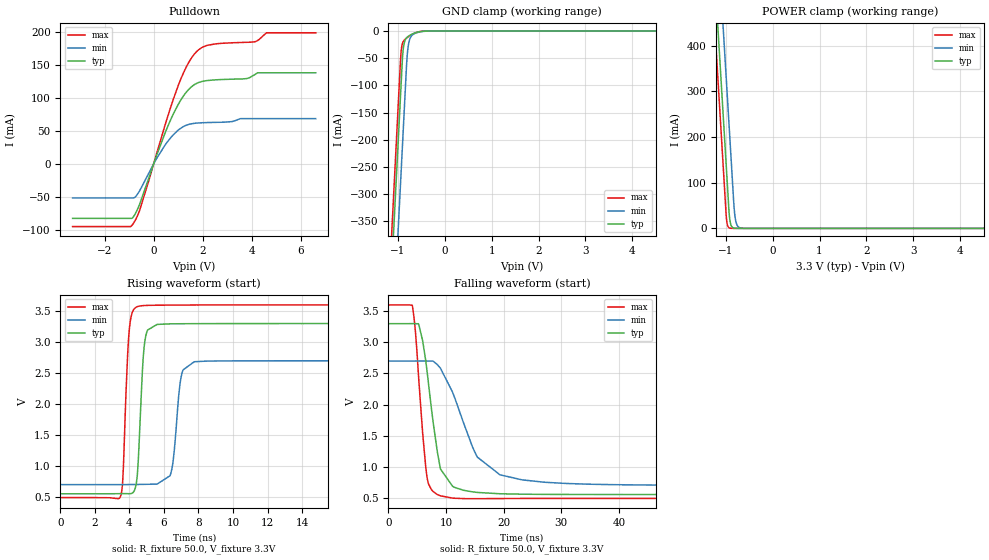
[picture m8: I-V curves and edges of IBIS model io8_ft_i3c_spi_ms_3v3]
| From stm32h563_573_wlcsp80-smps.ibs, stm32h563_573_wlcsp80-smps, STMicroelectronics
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[Model]   io8_ft_i3c_spi_ms_3v3
Model_type I/O_open_drain
Polarity   Non-Inverting
Enable   Active-Low
| CAP_THRESHOLD on pad IOFT is "UDTCAPC" :
| Rising=20.0% of vddiom   Falling=80.0% of vddiom
| C_comp min and max val. don't necessarily correlate with the min and max pvt
| but are the smallest and greatest pad capacitance found.
| var   typ   min   max
C_comp   3.95818pF  3.95032pF  4.00761pF
|C_comp_pulldown   3.95818pF  3.95032pF  4.00761pF
Vinl = 1.35V
Vinh = 1.8V
Vmeas = 1.65V   | Reference voltage for timing measurements
Cref  = 50.0pF   | Timing specification test load capacitance value
Rref  = 1.0MOhm   | Timing specification test load resistance value
Vref  = 1.815V   | Timing specification test load voltage
[Model Spec]
| TIME_THRESHOLD on pin ZII2CV11 is "CMOS" :
| Rising=40.0% of vdd   Falling=60.0% of vdd
Vinl 1.29880V 1.07480V 1.40680V
Vinh 1.77520V 1.49320V 1.89720V
| variable   typ   min   max
[Temperature Range] 25.0 125.0 -40.0
| variable   typ   min   max
[Voltage Range] 3.3V 2.7V 3.6V
| variable   typ   min   max
[POWER Clamp Reference] 3.3V 2.7V 3.6V
| variable   typ   min   max
[GND Clamp Reference] 0V 0V 0V
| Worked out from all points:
|   slope of the pulldown table from 0 to 0.495 V, typ, clamps not added: 10 ohm
|   GND clamp passes 1 mA (typ) near -0.52 V on its own axis
|   POWER clamp passes 1 mA (typ) near -0.84 V on its own axis
|   rising waveform, R_fixture 50.0, V_fixture 3.3V: 20-80 % time 285ps typ, 381ps min, 266ps max; typ from 0.556 V to 3.3 V
|   falling waveform, R_fixture 50.0, V_fixture 3.3V: 20-80 % time 2.35ns typ, 5.6ns min, 1.51ns max; typ from 3.3 V to 0.556 V
[POWER Clamp]
-3.3V     4.068A     4.259A     3.957A
-1.25V    582.8mA    774.2mA    471.5mA
-1.21V    514.8mA    706.2mA    403.5mA
-1.13V    378.8mA    570.2mA    267.5mA
-1.04V    225.8mA    417.2mA    114.5mA
-980mV    123.8mA    315.2mA    17.95mA
-920mV    26.3mA     213.2mA    906uA
-880mV    5.543mA    145.2mA    123.7uA
-810mV    363.5uA    33.6mA     3.798uA
-770mV    76.62uA    10.47mA    519.4nA
-690mV    3.409uA    1.017mA    10.46nA
6.6V      0A         0A         0A
[GND Clamp]
-3.3V     -4.13A     -4.291A    -4.063A
-1.25V    -644.7mA   -806.4mA   -578.1mA
-940mV    -117.7mA   -279.4mA   -51.06mA
-920mV    -83.75mA   -245.4mA   -31.43mA
-900mV    -50.5mA    -211.4mA   -23.14mA
-880mV    -31.27mA   -177.4mA   -19.1mA
-850mV    -18.68mA   -126.4mA   -15.73mA
-800mV    -11.46mA   -46.4mA    -12.03mA
-760mV    -8.752mA   -20.02mA   -9.606mA
-680mV    -5.122mA   -6.673mA   -5.579mA
-300mV    -5.379uA   -47.63uA   -852.7nA
6.6V      10.49nA    1.843uA    393.6pA
| variable   typ   min   max
[Pullup Reference] 3.3V 2.7V 3.6V
| variable   typ   min   max
[Pulldown Reference] 0V 0V 0V
[Pulldown]
-3.3V     -82.42mA   -51.49mA   -94.82mA
-850mV    -81.27mA   -51.49mA   -91.26mA
-580mV    -62.01mA   -41.36mA   -71.41mA
120mV     12.61mA    7.999mA    15.37mA
800mV     75.3mA     43.94mA    97.52mA
1.33V     108.3mA    58.37mA    146.5mA
1.84V     123.1mA    61.83mA    172.7mA
2.51V     126.9mA    62.7mA     181.3mA
3.78V     128.8mA    68.32mA    183.7mA
4.12V     134.9mA    68.32mA    184.6mA
4.59V     137.6mA    68.32mA    198mA
6.6V      137.6mA    68.32mA    198mA
[Ramp]
dV/dt_r 1.64663V/283.08572ps 1.19797V/378.54929ps 1.86385V/262.83539ps
dV/dt_f 1.64666V/2.32549ns 1.19801V/5.11685ns 1.86387V/1.50259ns
R_load = 50.0
| Removed startup time: 0s 0s 0s  .
| Removed end time: 34.4ns.
[Rising Waveform]
R_fixture   = 50.0
V_fixture   = 3.3V
V_fixture_min = 2.7V
V_fixture_max = 3.6V
0s        555.6mV    703.3mV    493.6mV
3.5ns     557mV      703.5mV    527.2mV
4ns       556.3mV    704.1mV    3.232V
4.5ns     1.04V      705.6mV    3.576V
4.9ns     3.032V     707.7mV    3.591V
5.6ns     3.286V     710.8mV    3.595V
6.4ns     3.295V     889.5mV    3.597V
7ns       3.297V     2.446V     3.598V
7.75ns    3.298V     2.684V     3.599V
34.4ns    3.3V       2.7V       3.6V
| Removed startup time: 0s 0s 0s  .
| Removed end time: 189.35ns.
[Falling Waveform]
R_fixture   = 50.0
V_fixture   = 3.3V
V_fixture_min = 2.7V
V_fixture_max = 3.6V
0s        3.3V       2.7V       3.6V
4.15ns    3.301V     2.7V       3.591V
5.25ns    3.292V     2.7V       2.436V
5.95ns    3.024V     2.7V       1.539V
6.9ns     2.387V     2.7V       747.4mV
9ns       982.7mV    2.589V     535.5mV
11.15ns   686.6mV    2.196V     498.3mV
15.45ns   588.9mV    1.156V     488.7mV
27.05ns   557.9mV    753.1mV    493.1mV
189.4ns   555.6mV    703.3mV    493.6mV
